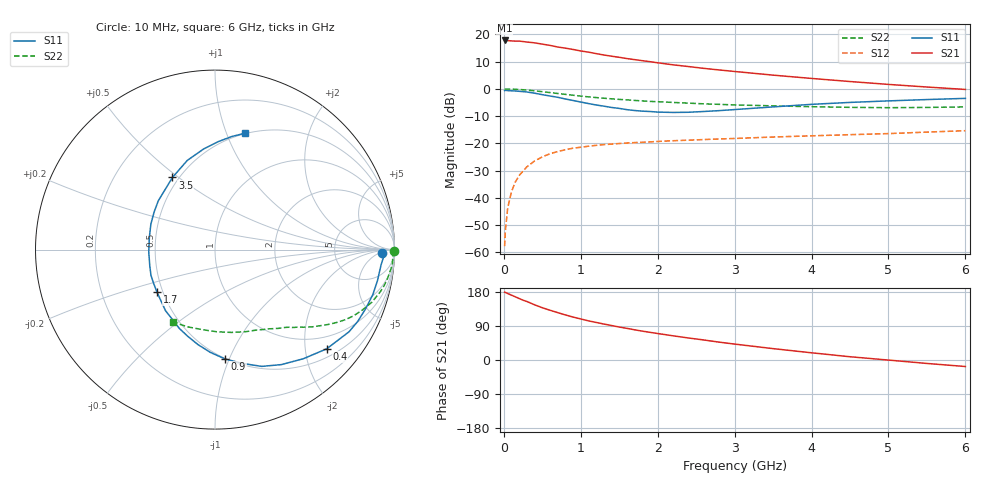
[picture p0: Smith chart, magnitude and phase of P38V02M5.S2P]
! SIEMENS Small Signal Semiconductors
! BFP181
! Si NPN RF Bipolar Junction Transistor in SOT143
! VCE = 8 V  IC = 2.5 mA
! Common Emitter S-Parameters:  March  1996
# GHz  S  MA  R  50
!  f  S11  S21  S12  S22
! GHz  MAG  ANG  MAG  ANG  MAG  ANG  MAG  ANG
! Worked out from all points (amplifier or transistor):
!   36 points, 10 MHz to 6 GHz, reference 50 ohm
!   highest |S21| = 17.8 dB at 10 MHz (marker M1)
!   |S21| within 3 dB of that: start of sweep to 836 MHz
!   unconditionally stable (mu >= 1): 2.396 GHz to end of sweep
!   at 250 MHz: K = 0.13, MSG = 23.8 dB, |S12| = -30.1 dB
!   at 1.4 GHz: K = 0.68, MSG = 16.1 dB, |S12| = -20.3 dB
!   at 6 GHz: K = 1.13, MAG = 5.4 dB, |S12| = -15.4 dB
!   S11 on the Smith chart (normalised r, x): 10 MHz: 25, -7; 400 MHz: 0.69, -2.47; 900 MHz: 0.50, -0.97; 1.7 GHz: 0.46, -0.26; 3.5 GHz: 0.46, +0.48; 6 GHz: 0.50, +1.16
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0.01  0.9284 -1.1  7.73 178.9  0.0013 82.1  0.9947 -0.5
0.02  0.9409 -2.3  7.704 178.4  0.0025 88.1  0.9894 -0.9
0.05  0.9293 -5.2  7.67 175.4  0.0065 86.4  0.9918 -2.5
0.1  0.9216 -10.8  7.588 171.1  0.0131 83.6  0.991 -5.0
0.2  0.9018 -21.4  7.526 162.2  0.0258 77.1  0.9737 -9.8
0.25  0.8903 -26.7  7.38 157.8  0.0311 74.7  0.9627 -12.2
0.4  0.8325 -41.6  6.987 145.6  0.0475 65.8  0.9214 -18.6
0.5  0.7823 -51.0  6.624 137.9  0.0565 60.1  0.8881 -22.2
0.6  0.7399 -60.0  6.277 131.3  0.0646 55.9  0.8554 -25.6
0.7  0.7008 -68.2  5.862 125.0  0.0708 52.1  0.8226 -28.4
0.8  0.652 -76.5  5.582 118.9  0.0764 48.6  0.7931 -30.7
0.9  0.612 -84.7  5.283 113.3  0.0817 45.6  0.764 -32.9
1.1  0.5375 -100.2  4.718 103.3  0.0887 40.4  0.7128 -36.7
1.4  0.4557 -121.4  3.974 91.0  0.097 34.8  0.6566 -41.2
1.7  0.4008 -143.7  3.439 79.7  0.1034 31.2  0.6139 -45.0
1.9  0.3844 -158.1  3.153 73.0  0.1064 29.1  0.5893 -47.3
2.2  0.3693 -178.0  2.761 63.8  0.1118 26.7  0.5637 -51.1
2.8  0.3988 148.2  2.224 47.1  0.1204 23.4  0.5199 -59.0
3.5  0.4667 120.5  1.786 30.0  0.1308 19.9  0.4882 -69.6
4.5  0.5644 96.4  1.364 8.6  0.1444 15.5  0.4581 -88.6
5.5  0.6367 81.6  1.081 -9.1  0.161 12.3  0.4565 -109.4
6  0.6692 75.6  0.976 -17.2  0.1708 10.2  0.4664 -120.2
